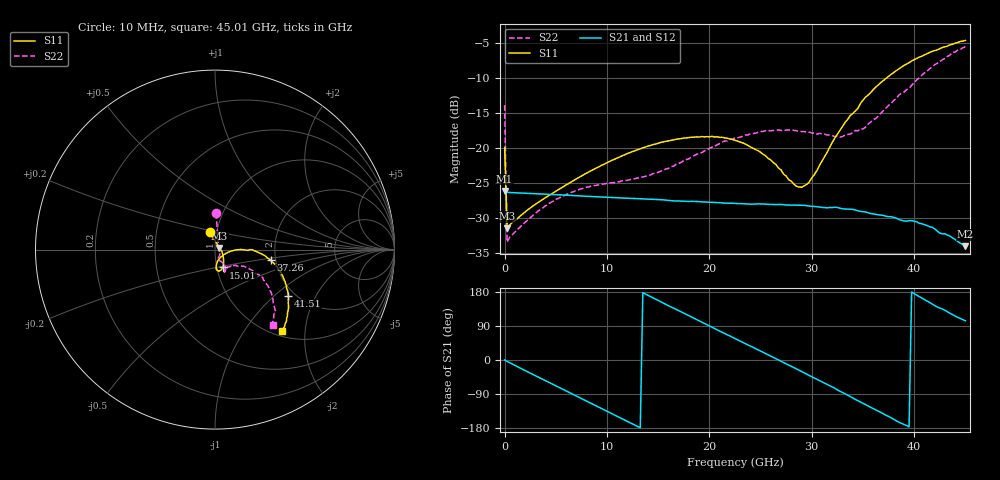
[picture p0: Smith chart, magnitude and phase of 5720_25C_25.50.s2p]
! Device:  ADRF5720
! Description: 0.5dB LSB GaAs MMIC 6-bit Digital Attenuator
! Frequency:  0.000009 -  40 GHz
! Ports:
!	RF1	= Port 1
!	RF2	= Port 2
! Vdd:  3.3 Volt
! Vss:  -3.3 Volt
! Control:  0/3.3 Volt
! State:  25.50 dB attenuation
! Data:  The device was measured using G-S-G Probes on a matrix board.
!  Data was collected using an calibrated 4 port network analyzer.
!  The reference plane for this measurement is at the launchers.
! Note:  Analog Devices supplies this data as a sample of measured data
!  for this product.  Your particular data for this product may vary.
!  Data was taken at 25 degrees C.
!  Analog Devices reserves the right to change this data at anytime.
# GHZ S DB R 45.0
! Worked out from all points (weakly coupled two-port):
!   181 points, 10 MHz to 45.01 GHz, reference 45 ohm
!   highest |S21| = -26.12 dB at 10 MHz (marker M1); lowest = -34.0 dB at 45.01 GHz (marker M2)
!   lowest |S11| = -31.5 dB at 260 MHz (marker M3), VSWR 1.05, Z = 47.3 + j0.871 ohm
!   |S11| at or under -10 dB: start of sweep to 37.28 GHz
!   |S22| runs from -33.4 to -5.5 dB; largest |S21 - S12| = 0.00015
!   S11 on the Smith chart (normalised r, x): 10 MHz: 0.93, +0.18; 15.01 GHz: 1.07, -0.22; 37.26 GHz: 1.88, -0.25; 41.51 GHz: 1.84, -1.24; 45.01 GHz: 1.09, -1.52
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0.01  -19.92 106.4  -26.12 0.1  -26.13 0.2  -13.85 88.2
0.26  -31.48 20.2  -26.32 -3.8  -26.33 -3.8  -33.44 22.5
1.76  -29.41 -3.2  -26.42 -24.3  -26.42 -24.3  -30.93 -16.8
4.01  -27.07 -23.2  -26.58 -54.7  -26.58 -54.7  -28.23 -47.1
7.76  -23.77 -44.0  -26.85 -104.9  -26.85 -104.9  -25.69 -71.0
15.01  -19.29 -66.5  -27.34 157.2  -27.34 157.2  -23.45 -66.5
15.26  -19.18 -67.2  -27.37 153.7  -27.37 153.7  -23.29 -65.8
20.26  -18.31 -79.6  -27.75 86.5  -27.75 86.5  -19.86 -58.8
22.76  -19.00 -85.3  -27.92 53.3  -27.92 53.3  -18.52 -60.6
25.51  -21.10 -84.9  -28.01 16.8  -28.00 16.8  -17.50 -64.9
28.51  -25.45 -58.0  -28.15 -23.6  -28.15 -23.6  -17.50 -67.8
29.51  -25.19 -35.0  -28.22 -37.6  -28.22 -37.6  -17.66 -66.2
30.26  -23.78 -18.5  -28.33 -47.7  -28.34 -47.6  -17.85 -65.7
32.76  -17.47 0.0  -28.59 -82.5  -28.58 -82.4  -18.43 -56.0
33.76  -15.35 -0.7  -28.72 -96.2  -28.72 -96.1  -17.98 -47.8
35.01  -13.13 -1.8  -29.07 -114.0  -29.08 -114.0  -17.27 -40.3
37.26  -10.02 -11.0  -29.73 -145.8  -29.73 -145.8  -14.28 -29.8
37.76  -9.44 -13.3  -29.80 -152.6  -29.80 -152.5  -13.62 -28.9
40.26  -7.18 -25.9  -30.54 171.1  -30.56 171.1  -10.25 -30.2
41.51  -6.31 -32.3  -31.22 152.1  -31.23 152.1  -8.65 -35.4
43.76  -5.15 -43.8  -32.83 119.5  -32.82 119.3  -6.27 -45.9
45.01  -4.60 -50.7  -34.01 103.6  -34.03 103.6  -5.50 -52.5
